TYPE ST_SafeControl :
STRUCT                      				
//	// Project 
	ComErr									AT%I*	:	BOOL;
	OtherErr								AT%I*	:	BOOL;
	InRun									AT%I*	:	BOOL;
	// CONTROL
	Run										AT%Q*	:	BOOL := TRUE;
	ErrAck									AT%Q*	:	BOOL;
	Restart									AT%Q*	:	BOOL;
END_STRUCT
END_TYPE
